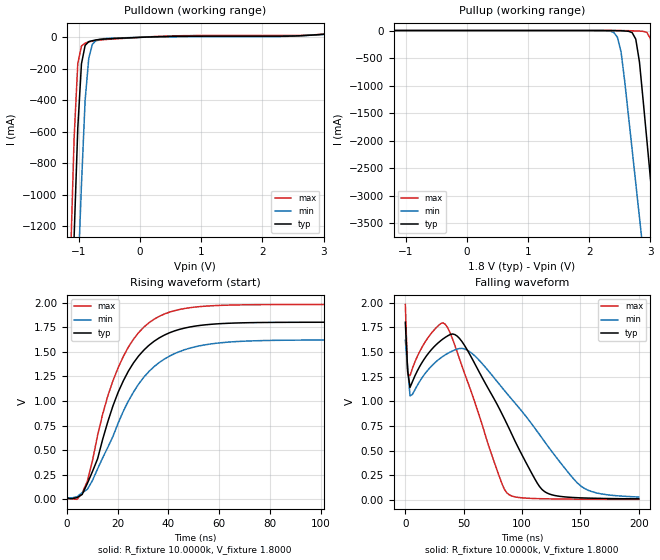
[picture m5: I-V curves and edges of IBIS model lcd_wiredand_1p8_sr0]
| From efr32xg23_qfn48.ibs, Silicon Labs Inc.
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|   Model lcd_wiredand_1p8_sr0
[Model]  lcd_wiredand_1p8_sr0
Model_type Output
Polarity   Inverting
Enable   Active-Low
C_comp   1.6300pF   1.4000pF   2.7000pF
[Temperature Range]   25.0000   0.1250k   -40.0000
[Pullup Reference]   1.8000V   1.6200V   1.9800V
[Pulldown Reference]   0.0V   0.0V   0.0V
[POWER Clamp Reference]   1.8000V   1.6200V   1.9800V
[GND Clamp Reference]   0.0V   0.0V   0.0V
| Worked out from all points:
|   slope of the pulldown table from 0 to 0.27 V, typ, clamps not added: 73.7 ohm
|   rising waveform, R_fixture 10.0000k, V_fixture 1.8000: 20-80 % time 16.4ns typ, 19.7ns min, 15ns max; typ from 0.011 V to 1.8 V
|   falling waveform, R_fixture 10.0000k, V_fixture 1.8000: 20-80 % time 47.1ns typ, 63.3ns min, 33.8ns max; typ from 1.8 V to 0.013 V
[Pulldown]
|Voltage   I(typ)   I(min)   I(max)
-1.8V     -9.882A    -9.584A    -10.33A
-1.14V    -1.981A    -2.781A    -1.427A
-1.08V    -1.267A    -2.165A    -640.1mA
-1.02V    -576.7mA   -1.55A     -166.6mA
-960mV    -168.5mA   -936.7mA   -54.94mA
-900mV    -51.19mA   -400.2mA   -36.82mA
-840mV    -27.26mA   -130.9mA   -28.21mA
-780mV    -21.22mA   -42.93mA   -24.16mA
-660mV    -13.38mA   -12.47mA   -17.5mA
540mV     5.932mA    3.464mA    9.194mA
2.7V      11.79mA    11.45mA    13.06mA
3.6V      40.81mA    35.67mA    44.95mA
[Pullup]
|Voltage   I(typ)   I(min)   I(max)
-1.8V     3.264nA    54.56nA    6.193nA
2.4V      -1.548mA   -34.03mA   -47.22uA
2.52V     -4.294mA   -392mA     -642.2uA
2.76V     -155.8mA   -2.773A    -7.422mA
2.82V     -568mA     -3.389A    -10.46mA
2.94V     -1.973A    -4.623A    -32.35mA
3V        -2.688A    -5.241A    -146.2mA
3.06V     -3.403A    -5.859A    -626.9mA
3.12V     -4.12A     -6.477A    -1.416A
3.24V     -5.555A    -7.713A    -3.027A
3.3V      -6.273A    -8.332A    -3.835A
3.6V      -9.867A    -11.43A    -7.885A
[Ramp]
| variable   typ   min   max
dV/dt_r  -0.1642m/68.8786p   -0.1873m/0.2201n   -0.1339m/36.8404p
dV/dt_f  1.0723/0.1024u   0.9530/0.1327u   1.1832/74.5294n
R_load = 10.0000k
[Rising Waveform]
R_fixture= 10.0000k
V_fixture= 1.8000
V_fixture_min= 1.6200
V_fixture_max= 1.9800
|time   V(typ)   V(min)   V(max)
0s        10.84mV    16.66mV    7.706mV
4.04ns    17.41mV    26.62mV    236.8uV
8.081ns   160.7mV    101.7mV    182.6mV
12.12ns   412.2mV    309.5mV    649.8mV
16.16ns   790.8mV    529.1mV    1.053V
22.22ns   1.203V     894.2mV    1.451V
30.3ns    1.516V     1.241V     1.75V
38.38ns   1.669V     1.425V     1.883V
68.69ns   1.794V     1.606V     1.976V
200ns     1.8V       1.62V      1.98V
[Falling Waveform]
R_fixture= 10.0000k
V_fixture= 1.8000
V_fixture_min= 1.6200
V_fixture_max= 1.9800
|time   V(typ)   V(min)   V(max)
0s        1.8V       1.62V      1.98V
2.02ns    1.306V     1.328V     1.278V
4.04ns    1.141V     1.055V     1.26V
18.18ns   1.461V     1.3V       1.623V
34.34ns   1.648V     1.471V     1.779V
48.48ns   1.605V     1.536V     1.358V
86.87ns   775.7mV    1.082V     74.85mV
121.2ns   73.05mV    560.7mV    13.17mV
153.5ns   21.64mV    118.2mV    9.222mV
200ns     12.9mV     31.64mV    8.019mV
